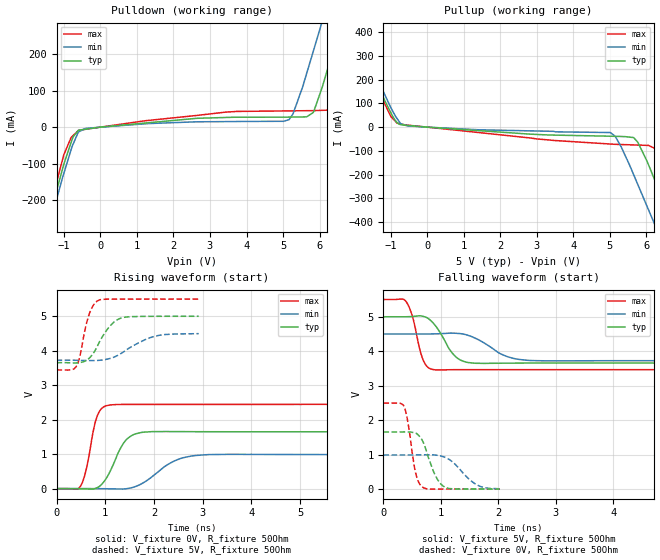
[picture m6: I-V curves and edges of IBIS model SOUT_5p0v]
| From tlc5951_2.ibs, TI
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|   sout_5p0v Model
[Model]   SOUT_5p0v
Model_type   Output
Polarity   Non-Inverting
Enable   Active-Low
Vmeas = 2.5
Vref = 2.5
Cref = 15pF
Rref = 50
|   typ   min   max
|   (nom PVT)   (Fast PVT)   (slow PVT)
|Average
C_comp   1.722e-12   1.053e-12   1.964e-12
|ON state : BUFFER OUTPUT TURNED HIGH
|C_comp   1.722e-12   1.053e-12   1.964e-12
|OFF state: BUFFER OUTPUT TURNED LOW
|C_comp   1.589e-12   1.369e-12   1.644e-12
| Where nom  PVT is Nominal Process,  5V,  65C
|   Fast PVT is Strong Process,   5.5V,  -40C
|   Slow PVT is Weak Process,   4.5V,  125C
[Voltage Range]   5   4.5   5.5
|Ambient Temperature   25   85   -40
|Junction Temperature
[Temperature Range]   65   125   -40
[Pullup Reference]   5   4.5   5.5
[Pulldown Reference]   0   0   0
[Power Clamp Reference]   5   4.5   5.5
[GND Clamp Reference]   0   0   0
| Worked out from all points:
|   slope of the pulldown table from 0 to 0.75 V, typ, clamps not added: 109 ohm
|   slope of the pullup table from 0 to 0.75 V, typ, clamps not added: 95.2 ohm
|   falling waveform, V_fixture 5V, R_fixture 50Ohm: 20-80 % time 301ps typ, 458ps min, 175ps max; typ from 5 V to 3.65 V
|   rising waveform, V_fixture 0V, R_fixture 50Ohm: 20-80 % time 343ps typ, 587ps min, 206ps max; typ from 0 V to 1.65 V
|   rising waveform, V_fixture 5V, R_fixture 50Ohm: 20-80 % time 352ps typ, 581ps min, 197ps max; typ from 3.65 V to 5 V
|   falling waveform, V_fixture 0V, R_fixture 50Ohm: 20-80 % time 223ps typ, 354ps min, 137ps max; typ from 1.66 V to 0 V
[Pulldown]
|   Voltage   I(typ)   I(min)   I(max)
-5V       -1.666A    -1.543A    -1.801A
-1.579V   -318.4mA   -335.7mA   -302.5mA
-1.36V    -232.4mA   -255.2mA   -213.7mA
-803.5mV  -42.59mA   -62.28mA   -28.88mA
-419mV    -5.85mA    -3.788mA   -6.066mA
5.165V    27.42mA    20.49mA    44.39mA
5.825V    39.75mA    206.1mA    45.08mA
6.075V    109.6mA    289.6mA    45.91mA
6.357V    206.1mA    382.5mA    47.7mA
6.54V     268.4mA    440.3mA    91.83mA
7.26V     531mA      668.4mA    357mA
10V       1.652A     1.658A     1.697A
[Pullup]
|   Voltage   I(typ)   I(min)   I(max)
-5V       1.614A     1.43A      1.949A
-2.437V   567.9mA    551.5mA    597.6mA
-1.953V   390.5mA    397.4mA    392.2mA
-996mV    60.56mA    82.02mA    45.36mA
-540.5mV  7.092mA    5.228mA    8.471mA
5.013V    -38.27mA   -22.74mA   -71.23mA
5.65V     -44.05mA   -200.7mA   -75.05mA
6.35V     -268.7mA   -455.4mA   -98.16mA
6.561V    -353.6mA   -529.7mA   -164.6mA
7.095V    -568.6mA   -716.5mA   -386.2mA
7.655V    -794.6mA   -913mA     -633.9mA
10V       -1.711A    -1.747A    -1.673A
[Ramp]
R_load = 50
|   typ   min   max
dV/dt_r   0.99324/3.44093e-10   0.592684/5.87128e-10   1.49689/2.09761e-10
dV/dt_f   0.807109/3.00876e-10   0.464821/4.57795e-10   1.2345/1.77108e-10
[Falling Waveform]
V_fixture = 5V
V_fixture_min = 4.5V
V_fixture_max = 5.5V
R_fixture = 50Ohm
|   Time   V(typ)   V(min)   V(max)
0s        5V         4.5V       5.5V
400ps     5V         4.5V       5.428V
500ps     5.007V     4.5V       5.037V
700ps     5.007V     4.499V     3.707V
900ps     4.75V      4.504V     3.459V
1.25ns    3.851V     4.521V     3.464V
1.625ns   3.649V     4.356V     3.465V
2.175ns   3.653V     3.832V     3.465V
2.85ns    3.656V     3.72V      3.464V
27.85ns   3.655V     3.725V     3.46V
[Rising Waveform]
V_fixture = 0V
V_fixture_min = 0V
V_fixture_max = 0V
R_fixture = 50Ohm
|   Time   V(typ)   V(min)   V(max)
0s        458.5pV    2.135nV    469.2pV
500ps     -3.006mV   641.5uV    88mV
600ps     -7.506mV   633.9uV    500.8mV
850ps     38.24mV    -1.254mV   2.156V
1.25ns    990.2mV    -9.512mV   2.44V
1.45ns    1.444V     977.7uV    2.443V
1.725ns   1.624V     125.8mV    2.443V
2.525ns   1.654V     862.9mV    2.442V
3.525ns   1.65V      994.9mV    2.443V
87.67ns   1.653V     987.7mV    2.471V
[Rising Waveform]
V_fixture = 5V
V_fixture_min = 4.5V
V_fixture_max = 5.5V
R_fixture = 50Ohm
|   Time   V(typ)   V(min)   V(max)
0s        3.655V     3.725V     3.442V
304ps     3.649V     3.725V     3.448V
424ps     3.648V     3.723V     3.587V
656ps     3.766V     3.715V     4.998V
752ps     3.92V      3.714V     5.312V
840ps     4.137V     3.719V     5.445V
1.088ns   4.703V     3.772V     5.497V
1.344ns   4.956V     3.938V     5.498V
2.016ns   4.999V     4.419V     5.499V
2.92ns    5V         4.496V     5.499V
[Falling Waveform]
V_fixture = 0V
V_fixture_min = 0V
V_fixture_max = 0V
R_fixture = 50Ohm
|   Time   V(typ)   V(min)   V(max)
0s        1.655V     987.8mV    2.495V
360ps     1.658V     987.7mV    2.402V
432ps     1.656V     988.2mV    1.877V
560ps     1.621V     990mV      473mV
616ps     1.551V     991.2mV    186.3mV
688ps     1.372V     993mV      46.51mV
880ps     473.5mV    989.1mV    -3.89mV
1.048ns   76.34mV    934.4mV    -537.6uV
1.592ns   88.74uV    153.8mV    629.8uV
2.024ns   208.7uV    6.851mV    577.9uV
